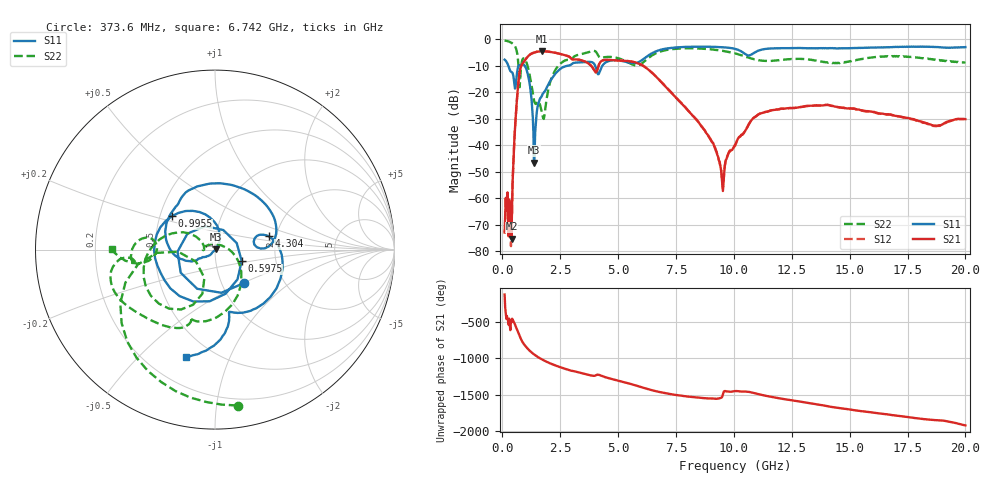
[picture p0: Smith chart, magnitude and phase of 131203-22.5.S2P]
!  2-Port S-parameters saved by WinCal
! VAR MeasName=S-Parameters (CALIBRATED_DATA) read from VNA (N5244A)
! VAR MeasDate=4/4/2013 3:58:20 PM
! VAR NAME=131203-22.5
! VAR FILENAME=131203-22.5.S2P
! VAR DATE=4/4/2013 3:58:20 PM
! VAR PHYS_PORTS=1,2
# Hz S MA R 50
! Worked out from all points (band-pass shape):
!   801 points, 100 MHz to 20 GHz, reference 50 ohm
!   highest |S21| = -4.47 dB at 1.717 GHz (marker M1); lowest = -75.2 dB at 398.5 MHz (marker M2)
!   |S21| within 3 dB of the highest: 1.008 GHz to 3.023 GHz (2.015 GHz wide, 100 % of centre)
!   lowest |S11| = -46.4 dB at 1.369 GHz (marker M3), VSWR 1.01, Z = 50.5 + j0.141 ohm
!   |S11| at or under -10 dB: 269 MHz to 702.9 MHz (434 MHz wide, 89.3 % of centre); 972.9 MHz to 2.77 GHz (1.797 GHz wide, 96 % of centre); 4.013 GHz to 4.317 GHz (304.5 MHz wide, 7.31 % of centre)
!   |S22| runs from -30.0 to -0.4 dB; largest |S21 - S12| = 0.0032
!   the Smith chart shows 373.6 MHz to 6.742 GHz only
!   S11 on the Smith chart (normalised r, x): 373.6 MHz: 1.27, -0.51; 597.5 MHz: 1.34, -0.18; 995.5 MHz: 0.58, +0.24; 4.304 GHz: 1.83, +0.30; 6.742 GHz: 0.36, -0.70
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1e8  0.4156 144.7  0.0002274 -122.5  0.0002311 15.0  0.9571 -22.2
3.73625e8  0.2464 -49.4  0.0003059 -116.3  0.0001257 -79.3  0.8777 -81.8
3.985e8  0.243 -81.7  0.0001748 -143.9  0.0005372 -141.5  0.8645 -87.5
5.975e8  0.162 -23.3  0.04529 151.2  0.04535 151.4  0.6625 -141.8
7.71625e8  0.3291 -148.6  0.2706 11.8  0.2711 11.9  0.1682 -110.6
9.955e8  0.3036 142.3  0.4162 -109.3  0.4169 -109.2  0.4098 -165.8
1.169625e9  0.1564 91.8  0.5077 -169.6  0.5092 -169.5  0.2271 155.1
1.368625e9  0.004762 17.0  0.5629 136.2  0.5649 136.2  0.0722 156.1
1.716875e9  0.08749 -148.0  0.5976 65.8  0.5996 65.8  0.04034 132.4
2.09e9  0.1705 -158.4  0.5791 9.3  0.5805 9.2  0.1685 -34.2
2.5875e9  0.2946 160.3  0.521 -49.4  0.5216 -49.5  0.3737 -87.6
3.43325e9  0.3713 77.1  0.4015 -122.5  0.4018 -122.4  0.5314 -132.5
4.303875e9  0.3099 13.8  0.3976 -161.7  0.3989 -161.8  0.4518 -170.7
5.448125e9  0.3672 -73.0  0.3896 98.2  0.391 98.3  0.3659 170.0
6.741625e9  0.6185 -105.2  0.1792 -17.5  0.1807 -17.6  0.5742 179.8
8.80625e9  0.7293 -173.5  0.01713 -107.0  0.01737 -107.6  0.662 128.0
9.50275e9  0.7147 169.8  0.001728 -79.5  0.002004 -83.6  0.6102 113.7
1.005e10  0.6658 156.3  0.01028 -8.4  0.009728 -11.8  0.5452 104.2
1.111962e10  0.6284 158.7  0.0396 -54.7  0.04008 -55.4  0.4036 100.2
1.338325e10  0.683 124.7  0.05617 -179.9  0.05588 179.5  0.4082 90.7
1.669162e10  0.7147 92.4  0.03873 29.2  0.0382 28.6  0.4764 80.8
2e10  0.7164 57.9  0.03131 -120.2  0.03114 -120.7  0.3679 59.2
